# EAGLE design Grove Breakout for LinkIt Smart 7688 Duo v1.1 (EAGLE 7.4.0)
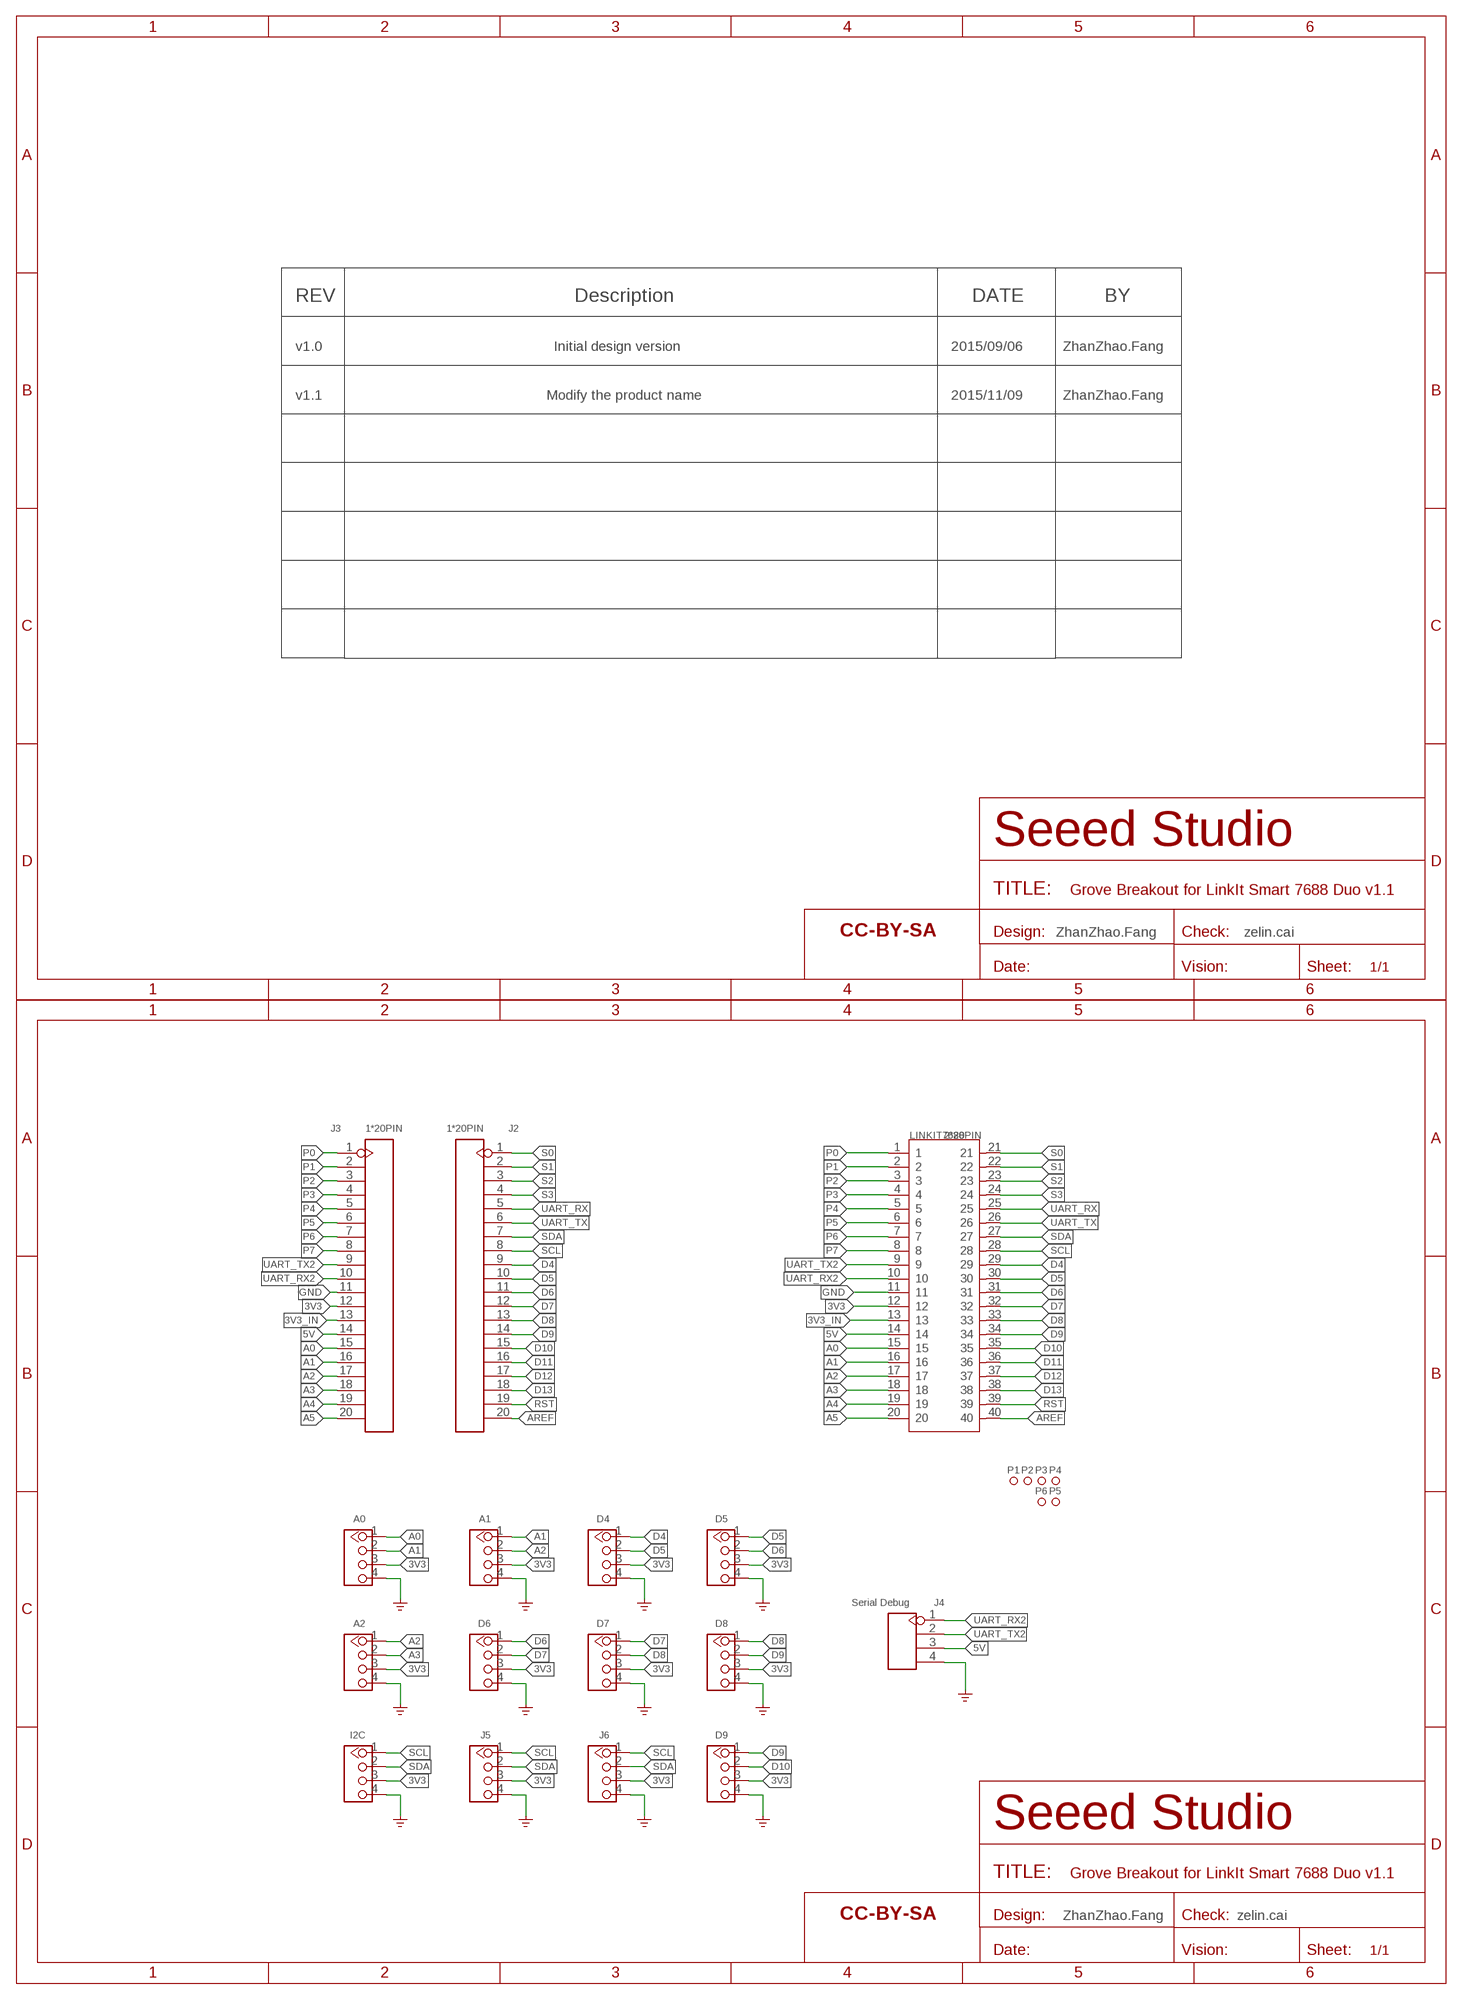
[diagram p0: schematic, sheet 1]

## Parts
A0  320110033  GROVE-CONNECTOR-DIP-2.0  [HW4-2.0]
A1  320110033  GROVE-CONNECTOR-DIP-2.0  [HW4-2.0]
A2  320110033  GROVE-CONNECTOR-DIP-2.0  [HW4-2.0]
D4  320110033  GROVE-CONNECTOR-DIP-2.0  [HW4-2.0]
D5  320110033  GROVE-CONNECTOR-DIP-2.0  [HW4-2.0]
D6  320110033  GROVE-CONNECTOR-DIP-2.0  [HW4-2.0]
D7  320110033  GROVE-CONNECTOR-DIP-2.0  [HW4-2.0]
D8  320110033  GROVE-CONNECTOR-DIP-2.0  [HW4-2.0]
D9  320110033  GROVE-CONNECTOR-DIP-2.0  [HW4-2.0]
FR1  DNP  SEEEDSTUDIO-OPEN-SCH-FRAME  [SEEEDSTUDIO-PCB-FRAME]
FR2  DNP  SEEEDSTUDIO-OPEN-SCH-FRAME  [SEEEDSTUDIO-PCB-FRAME]
I2C  320110033  GROVE-CONNECTOR-DIP-2.0  [HW4-2.0]
J2  1*20PIN  HEADER-20P-2.54  [H20-2.54]
J3  1*20PIN  HEADER-20P-2.54  [H20-2.54]
J4  Serial Debug  HEADER-4P-80/40MIL  [H4-2.54-C80D40MIL]
J5  320110033  GROVE-CONNECTOR-DIP-2.0  [HW4-2.0]
J6  320110033  GROVE-CONNECTOR-DIP-2.0  [HW4-2.0]
LINKIT7688  2*20PIN  LINKIT-7688-DUO  [HEADER-2X20P-2.54-65/35MIL]
P1  MARK-1.0'ANNULAR'  [ROUND-MARK-1.0]
P2  MARK-1.0'ANNULAR'  [ROUND-MARK-1.0]
P3  MARK-1.0'ANNULAR'  [ROUND-MARK-1.0]
P4  MARK-1.0'ANNULAR'  [ROUND-MARK-1.0]
P5  MARK-1.0'ANNULAR'  [ROUND-MARK-1.0]
P6  MARK-1.0'ANNULAR'  [ROUND-MARK-1.0]

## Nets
3V3: A0.3 A1.3 A2.3 D4.3 D5.3 D6.3 D7.3 D8.3 D9.3 I2C.3 J3.12 J5.3 J6.3 LINKIT7688.12
3V3_IN: J3.13 LINKIT7688.13
5V: J3.14 J4.3 LINKIT7688.14
A0: A0.1 J3.15 LINKIT7688.15
A1: A0.2 A1.1 J3.16 LINKIT7688.16
A2: A1.2 A2.1 J3.17 LINKIT7688.17
A3: A2.2 J3.18 LINKIT7688.18
A4: J3.19 LINKIT7688.19
A5: J3.20 LINKIT7688.20
AREF: J2.20 LINKIT7688.40
D4: D4.1 J2.9 LINKIT7688.29
D5: D4.2 D5.1 J2.10 LINKIT7688.30
D6: D5.2 D6.1 J2.11 LINKIT7688.31
D7: D6.2 D7.1 J2.12 LINKIT7688.32
D8: D7.2 D8.1 J2.13 LINKIT7688.33
D9: D8.2 D9.1 J2.14 LINKIT7688.34
D10: D9.2 J2.15 LINKIT7688.35
D11: J2.16 LINKIT7688.36
D12: J2.17 LINKIT7688.37
D13: J2.18 LINKIT7688.38
GND: A0.4 A1.4 A2.4 D4.4 D5.4 D6.4 D7.4 D8.4 D9.4 I2C.4 J3.11 J4.4 J5.4 J6.4 LINKIT7688.11 ; supply symbol labelled GND_POWER
P0: J3.1 LINKIT7688.1
P1: J3.2 LINKIT7688.2
P2: J3.3 LINKIT7688.3
P3: J3.4 LINKIT7688.4
P4: J3.5 LINKIT7688.5
P5: J3.6 LINKIT7688.6
P6: J3.7 LINKIT7688.7
P7: J3.8 LINKIT7688.8
RST: J2.19 LINKIT7688.39
S0: J2.1 LINKIT7688.21
S1: J2.2 LINKIT7688.22
S2: J2.3 LINKIT7688.23
S3: J2.4 LINKIT7688.24
SCL: I2C.1 J2.8 J5.1 J6.1 LINKIT7688.28
SDA: I2C.2 J2.7 J5.2 J6.2 LINKIT7688.27
UART_RX: J2.5 LINKIT7688.25
UART_RX2: J3.10 J4.1 LINKIT7688.10
UART_TX: J2.6 LINKIT7688.26
UART_TX2: J3.9 J4.2 LINKIT7688.9

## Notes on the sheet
- REV | Description | DATE | BY
- v1.0 | Initial design version | 2015/09/06 | ZhanZhao.Fang
- v1.1 | Modify the product name | 2015/11/09 | ZhanZhao.Fang
- ZhanZhao.Fang | zelin.cai
- ZhanZhao.Fang | zelin.cai

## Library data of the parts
A0 A1 A2 D4-D9 I2C J5 J6 = Connector-new:GROVE-CONNECTOR-DIP: 4P-2.0:320110033;4P-2.0-90D:320110034
FR1 FR2 = moudle-new:SEEEDSTUDIO-OPEN-SCH-FRAME
J2 J3 = Connector-new:HEADER-20P
J4 = Connector-new:HEADER-4P
LINKIT7688 = template:LINKIT-7688-DUO
P1-P6 = Discrete-new:MARK-1.0; PARTNO: DNP

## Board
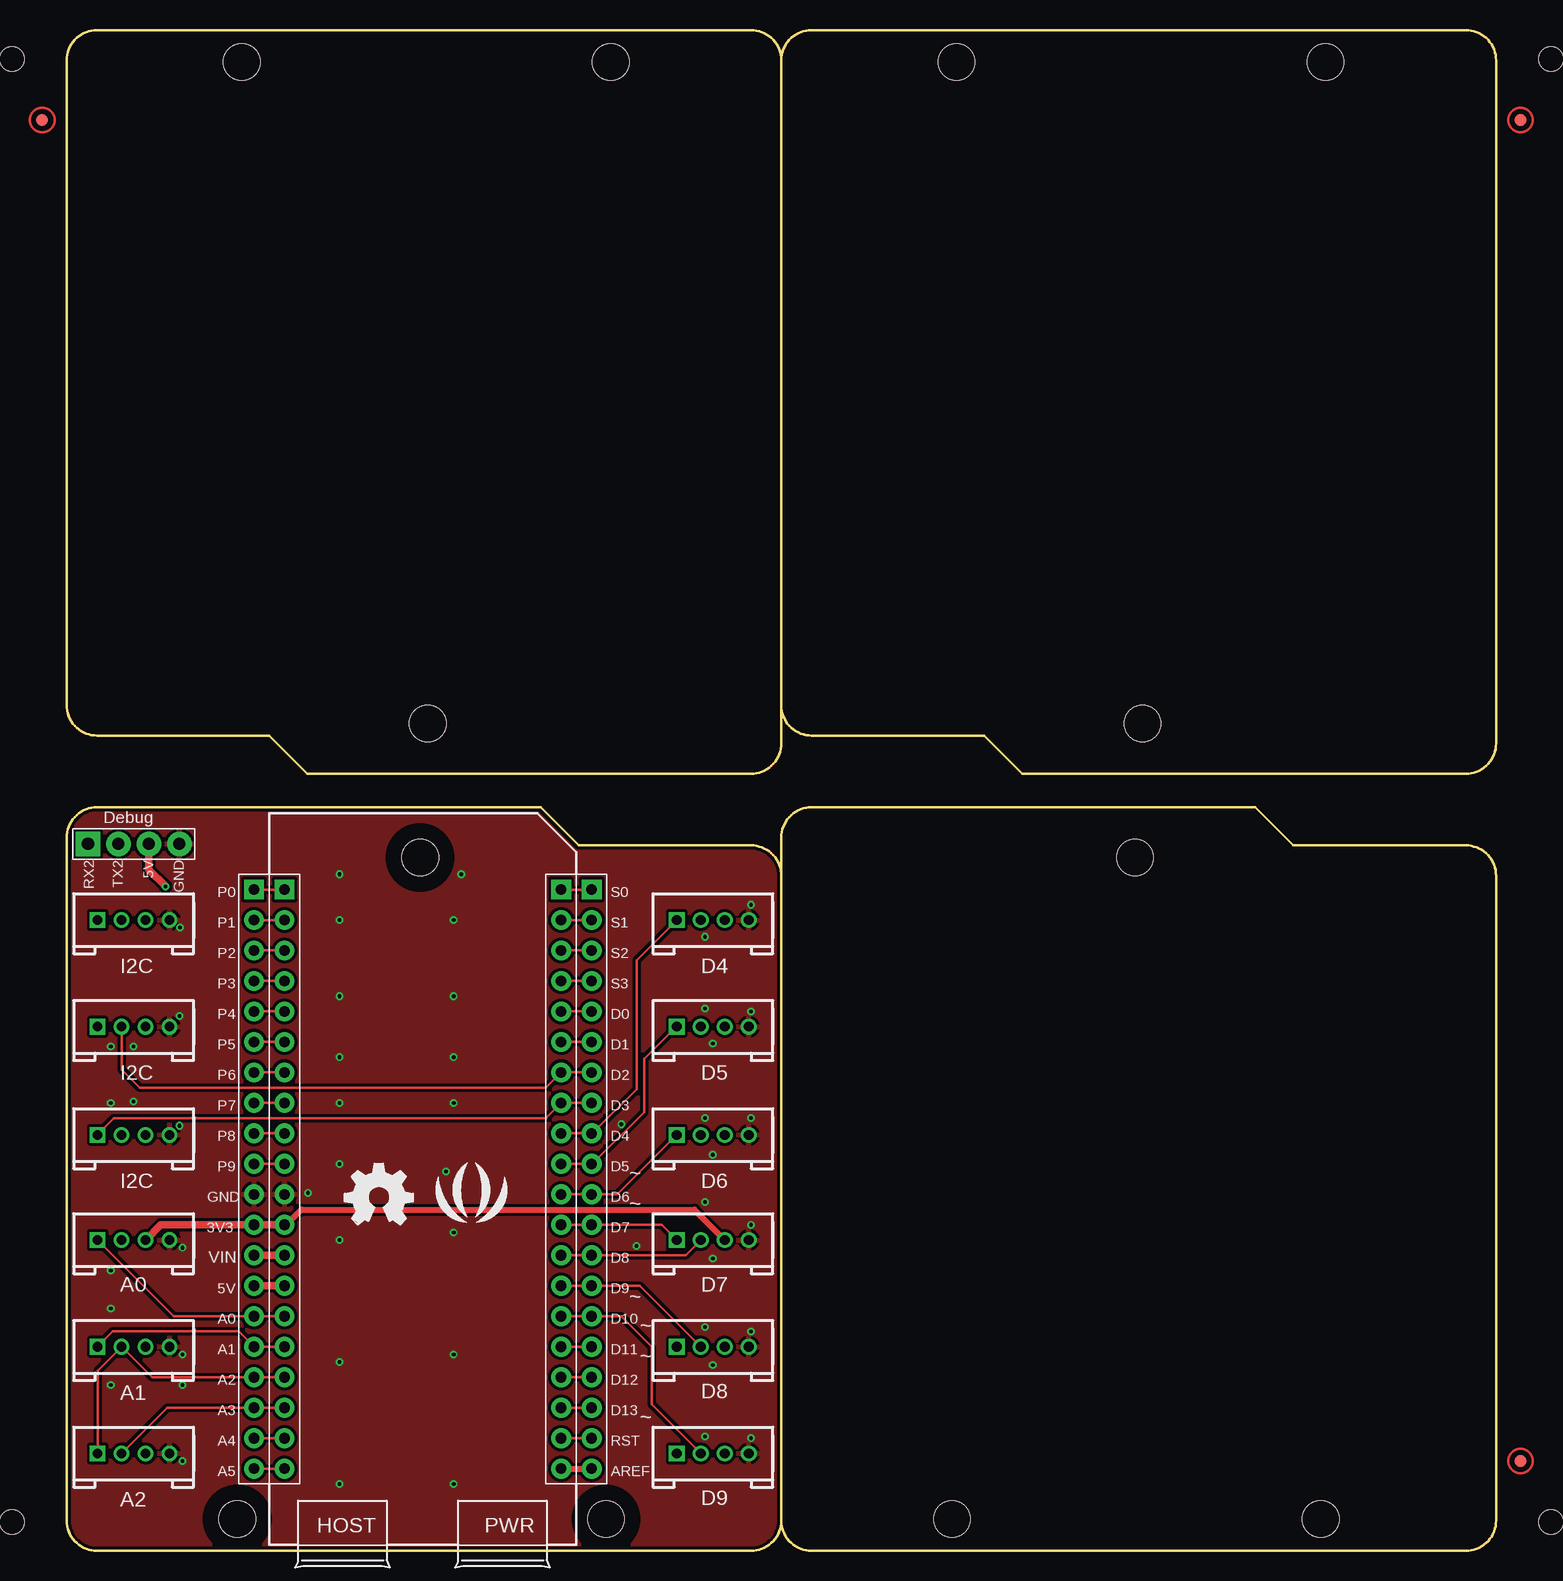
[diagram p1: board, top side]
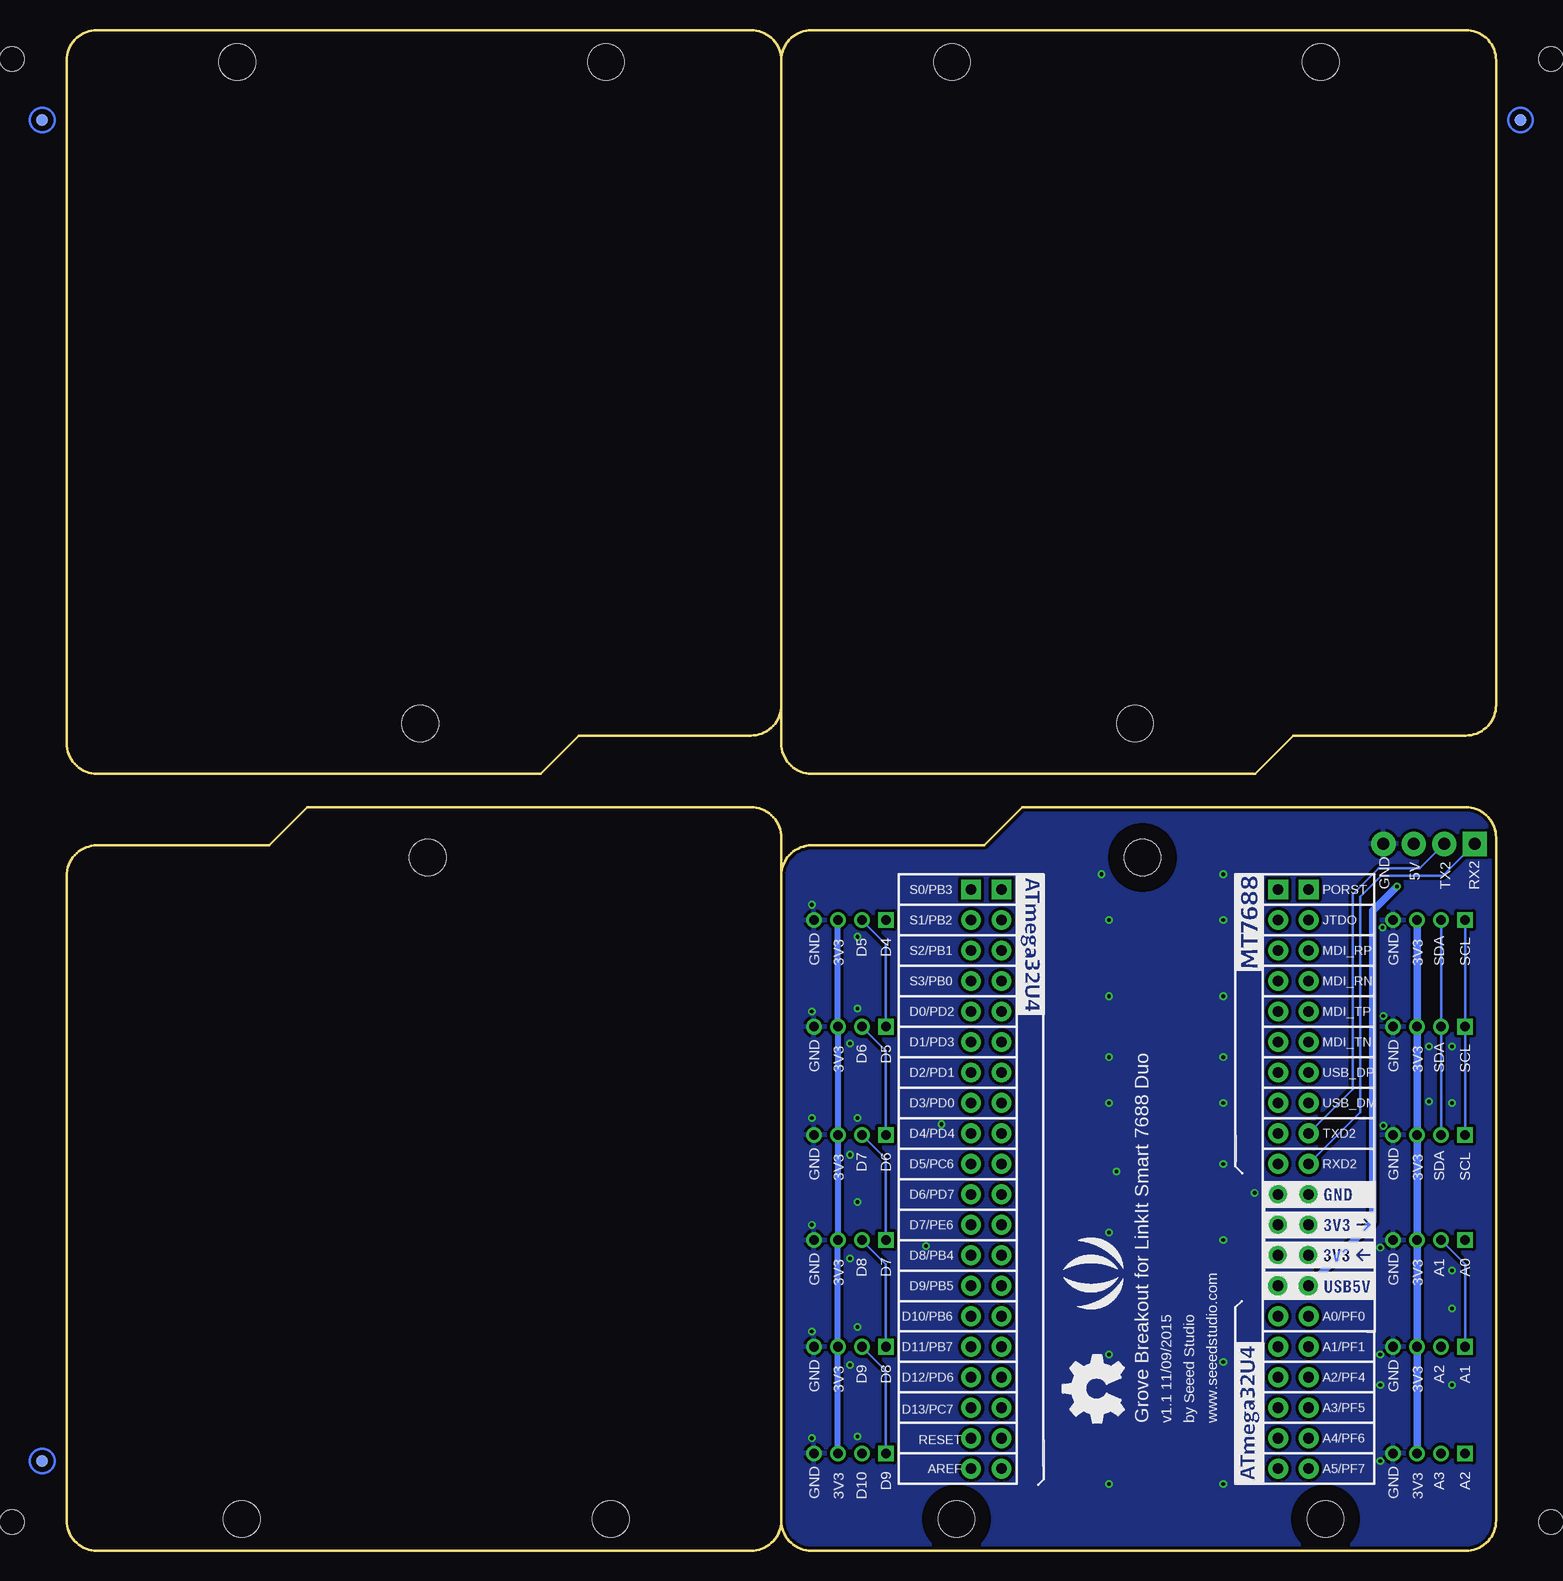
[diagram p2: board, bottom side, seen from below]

Size 119.13 x 126.75 mm. Coordinates in mm from the lower left corner, seen from the top.
Outline: 59.56,56.26 59.56,2.54
Outline: 59.56,2.54 arc-90 57.02,0 2.54,0 arc-90 0,2.54 0,59.44 arc-90 2.54,61.98 39.5,61.98 42.67,58.8 57.02,58.8 arc-90 59.56,56.26
Outline: 59.56,56.26 59.56,59.44 arc-90 62.1,61.98 99.06,61.98 102.23,58.8 116.59,58.8 arc-90 119.13,56.26 119.13,2.54 arc-90 116.59,0 62.1,0 arc-90 59.56,2.54
Outline: 59.56,70.48 59.56,124.21
Outline: 59.56,124.21 arc-90 62.1,126.75 116.59,126.75 arc-90 119.13,124.21 119.13,67.31 arc-90 116.59,64.77 79.63,64.77 76.45,67.94 62.1,67.94 arc-90 59.56,70.48
Outline: 59.56,70.48 59.56,67.31 arc-90 57.02,64.77 20.07,64.77 16.89,67.94 2.54,67.94 arc-90 0,70.48 0,124.21 arc-90 2.54,126.75 57.02,126.75 arc-90 59.56,124.21
Copper layers (1*16): Top 0.035mm / dielectric 1.5mm / Bottom 0.035mm
Design rules "SeeedStudio_2layer_DRU_no_angle_20140221 *": minimum track width 6mil, minimum drill 12mil, track to track 6mil, track to pad 6mil, pad to pad 6mil, via to via 6mil, smd to smd 0mil, copper to edge 10mil, drill to drill 10mil, minimum pad ring 10mil, minimum via ring 6mil, stop-mask expansion 2mil, vias tented up to drill 25mil, thermal gap 10mil
Holes 3.05 mm at 29.46,57.79 14.22,2.67 44.96,2.67 89.03,57.79 73.79,2.67 104.52,2.67 89.66,68.96 104.9,124.08 74.17,124.08 30.1,68.96 45.34,124.08 14.61,124.08
Holes 2.03 mm at -4.57,124.33 -4.57,2.41 123.7,124.33 123.7,2.41
tRestrict: area 27,55.3 to 32,60.3; area 11.7,0.2 to 16.7,5.2; area 42.5,0.2 to 47.5,5.2
bRestrict: area 27,55.3 to 32,60.3; area 11.7,0.2 to 16.7,5.2; area 42.5,0.2 to 47.5,5.2

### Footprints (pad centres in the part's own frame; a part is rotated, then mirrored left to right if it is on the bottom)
HW4-2.0 = drill 0.8 pad 1.27 square: 1 -3,0 | drill 0.8 pad 1.27: 2 -1,0; 3 1,0; 4 3,0
H20-2.54 = drill 0.889 pad 1.651 square: 1 0,-24.13 | drill 0.889 pad 1.651: 2 0,-21.59; 3 0,-19.05; 4 0,-16.51; 5 0,-13.97; 6 0,-11.43; 7 0,-8.89; 8 0,-6.35; 9 0,-3.81; 10 0,-1.27; 11 0,1.27; 12 0,3.81; 13 0,6.35; 14 0,8.89; 15 0,11.43; 16 0,13.97; 17 0,16.51; 18 0,19.05; 19 0,21.59; 20 0,24.13
H4-2.54-C80D40MIL = drill 1.016 pad 2.032 square: 1 0,3.81 | drill 1.016 pad 2.032: 2 0,1.27; 3 0,-1.27; 4 0,-3.81
HEADER-2X20P-2.54-65/35MIL = drill 0.889 pad 1.651 square: 1 0,24.13; 21 23.05,24.13 | drill 0.889 pad 1.651: 2 0,21.59; 3 0,19.05; 4 0,16.51; 5 0,13.97; 6 0,11.43; 7 0,8.89; 8 0,6.35; 9 0,3.81; 10 0,1.27; 11 0,-1.27; 12 0,-3.81; 13 0,-6.35; 14 0,-8.89; 15 0,-11.43; 16 0,-13.97; 17 0,-16.51; 18 0,-19.05; 19 0,-21.59; 20 0,-24.13; 22 23.05,21.59; 23 23.05,19.05; 24 23.05,16.51; 25 23.05,13.97; 26 23.05,11.43; 27 23.05,8.89; 28 23.05,6.35; 29 23.05,3.81; 30 23.05,1.27; 31 23.05,-1.27; 32 23.05,-3.81; 33 23.05,-6.35; 34 23.05,-8.89; 35 23.05,-11.43; 36 23.05,-13.97; 37 23.05,-16.51; 38 23.05,-19.05; 39 23.05,-21.59; 40 23.05,-24.13
ROUND-MARK-1.0 = smd 1.016 x 1.016: P$1 0,0

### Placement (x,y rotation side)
A0  5.59,25.91 0 top
A1  5.59,17.02 0 top
A2  5.59,8.13 0 top
D4  53.85,52.58 0 top
D5  53.85,43.69 0 top
D6  53.85,34.67 0 top
D7  53.85,25.91 0 top
D8  53.85,17.02 0 top
D9  53.85,8.13 0 top
FR1  not placed on the board
FR2  not placed on the board
I2C  5.59,52.58 0 top
J2  43.75,30.99 180 top
J3  15.62,30.99 180 top
J4  5.59,58.93 90 top
J5  5.59,43.69 0 top
J6  5.59,34.67 0 top
LINKIT7688  18.16,30.99 0 top
P1  -2.03,119.25 0 top
P2  -2.03,119.25 0 bottom
P3  121.16,119.25 0 top
P4  121.16,119.25 0 bottom
P5  121.16,7.49 0 top
P6  121.16,7.49 0 bottom
U$14  [OSHW_FILLX200_NOTEXT]  31.01,10.68 90 bottom
U$15  [SEEED-SILK-280*268MIL]  32.77,23.11 90 bottom
U$16  [OSHW_FILLX200_NOTEXT]  23.19,27.2 0 top
U$17  [SEEED-SILK-280*268MIL]  33.73,29.08 0 top

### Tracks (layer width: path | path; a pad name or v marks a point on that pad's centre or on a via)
3V3
  Top 0.508: LINKIT7688.12 18.29,27.18 19.56,28.45 52.31,28.45 D7.3
  Top 0.61: A0.3 7.86,27.18 J3.12 LINKIT7688.12
  Bottom 0.508: D9.3 D8.3 D7.3 D6.3 D5.3 D4.3
  Bottom 0.61: A2.3 A1.3 A0.3 J6.3 J5.3 I2C.3
3V3_IN
  Top 0.61: J3.13 LINKIT7688.13
5V  (via drill 0.3 pad 0.64)
  Top 0.61: J3.14 LINKIT7688.14 | J4.3 6.86,56.77 v8.26,55.37
  Bottom 0.61: v8.26,55.37 10.29,53.34 10.29,27.43 J3.14
A0
  Top 0.203: A0.1 8.94,19.56 J3.15 LINKIT7688.15
A1
  Top 0.203: LINKIT7688.16 J3.16 14.35,18.29 3.86,18.29 A1.1
  Bottom 0.203: A1.1 2.59,23.91 A0.2
A2
  Top 0.203: A2.1 2.59,15.02 A1.2 7.13,14.48 J3.17 LINKIT7688.17
A3
  Top 0.203: A2.2 8.4,11.94 J3.18 LINKIT7688.18
A4
  Top 0.203: J3.19 LINKIT7688.19
A5
  Top 0.203: J3.20 LINKIT7688.20
AREF
  Top 0.508: LINKIT7688.40 J2.20
D4
  Top 0.203: LINKIT7688.29 J2.9 43.81,34.8 47.5,38.48 47.5,49.23 D4.1
D5
  Top 0.203: LINKIT7688.30 J2.10 43.81,32.26 48.13,36.58 48.13,41.02 50.8,43.69 D5.1
  Bottom 0.203: D5.1 50.85,50.58 D4.2
D6
  Top 0.203: LINKIT7688.31 J2.11 45.9,29.72 D6.1
  Bottom 0.203: D6.1 50.85,41.69 D5.2
D7
  Top 0.203: LINKIT7688.32 J2.12 49.58,27.18 D7.1
  Bottom 0.203: D7.1 50.85,32.67 D6.2
D8
  Top 0.203: LINKIT7688.33 J2.13 51.58,24.64 D7.2
  Bottom 0.203: D8.1 50.85,23.91 D7.2
D9
  Top 0.203: LINKIT7688.34 J2.14 47.77,22.1 D8.2
  Bottom 0.203: D9.1 50.85,15.02 D8.2
D10
  Top 0.203: LINKIT7688.35 J2.15 46.23,19.56 48.77,17.02 48.77,12.21 D9.2
D11
  Top 0.203: LINKIT7688.36 J2.16
D12
  Top 0.203: LINKIT7688.37 J2.17
D13
  Top 0.203: LINKIT7688.38 J2.18
GND  (via drill 0.3 pad 0.64)
  other vias: 9.46,51.94 9.4,44.58 9.4,35.43 9.65,25.27 9.65,16.38 9.65,7.49 20.12,29.84 57.02,9.4 57.02,18.29 57.02,27.18 57.02,36.07 57.02,44.96 57.02,53.85 22.73,5.59 32.26,5.59 32.26,16.38 22.73,15.75 22.73,25.91 32.26,26.54 32.26,41.15 22.73,41.15 22.73,56.39 32.89,56.39 31.62,31.62 22.73,32.26 22.73,46.23 32.26,46.23 22.73,37.34 32.26,37.34 3.68,13.84 9.65,13.84 22.73,52.58 32.26,52.58 46.23,35.56 47.5,25.4 53.21,51.18 53.21,45.21 53.85,42.29 53.21,36.07 53.85,33.02 53.21,29.08 53.85,24.38 53.21,18.67 53.85,15.49 53.21,9.52 3.68,20.19 3.68,23.37 3.68,37.34 3.68,42.04 5.59,42.04 5.59,37.47
  pour Bottom (isolate 0.254): -0.63,62.74 60.2,62.74 60.2,-0.76 -0.63,-0.76
  pour Top (isolate 0.254): -0.63,62.74 60.2,62.74 60.2,-0.76 -0.63,-0.76
P0
  Top 0.203: J3.1 LINKIT7688.1
P1
  Top 0.203: J3.2 LINKIT7688.2
P2
  Top 0.203: J3.3 LINKIT7688.3
P3
  Top 0.203: J3.4 LINKIT7688.4
P4
  Top 0.203: J3.5 LINKIT7688.5
P5
  Top 0.203: J3.6 LINKIT7688.6
P6
  Top 0.203: J3.7 LINKIT7688.7
P7
  Top 0.203: J3.8 LINKIT7688.8
RST
  Top 0.203: LINKIT7688.39 J2.19
S0
  Top 0.203: LINKIT7688.21 J2.1
S1
  Top 0.203: LINKIT7688.22 J2.2
S2
  Top 0.203: J2.3 LINKIT7688.23
S3
  Top 0.203: LINKIT7688.24 J2.4
SCL
  Top 0.203: J6.1 2.59,34.72 3.94,36.07 39.94,36.07 LINKIT7688.28 J2.8
  Bottom 0.203: J6.1 J5.1 I2C.1
SDA
  Top 0.203: J5.2 4.59,40.12 6.1,38.61 39.94,38.61 LINKIT7688.27 J2.7
  Bottom 0.203: J6.2 J5.2 I2C.2
UART_RX
  Top 0.203: LINKIT7688.25 J2.5
UART_RX2
  Top 0.203: LINKIT7688.10 J3.10
  Bottom 0.203: J3.10 11.3,36.58 11.3,54.53 9.58,56.26 4.45,56.26 J4.1
UART_TX
  Top 0.203: LINKIT7688.26 J2.6
UART_TX2
  Top 0.203: J3.9 LINKIT7688.9
  Bottom 0.203: J3.9 11.94,38.48 11.94,54.74 9.78,56.9 6.35,56.9 J4.2

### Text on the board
tPlace: Debug | RX2 | TX2 | 5V | GND | P0 | S0 | P1 | S1 | P2 | S2 | P3 | S3 | P4 | D0 | P5 | D1 | I2C | P6 | D2 | P7 | D3 | P8 | D4 | P9 | D5 | I2C | ~ | GND | D6 | ~ | 3V3 | D7 | VIN | D8 | 5V | D9 | ~ | A0 | D10 | ~ | A1 | D11 | ~ | A2 | D12 | A3 | D13 | ~ | A4 | RST | A5 | AREF | HOST | PWR
bPlace: RX2 | TX2 | 5V | GND | PORST | S0/PB3 | JTDO | S1/PB2 | MDI_RP | S2/PB1 | D4 | D5 | SCL | SDA | 3V3 | GND | 3V3 | GND | MDI_RN | S3/PB0 | MDI_TP | D0/PD2 | MDI_TN | D1/PD3 | D5 | D6 | SCL | SDA | 3V3 | GND | USB_DP | D2/PD1 | 3V3 | GND | USB_DM | D3/PD0 | TXD2 | D4/PD4 | RXD2 | D5/PC6 | D6 | D7 | SCL | SDA | 3V3 | GND | 3V3 | GND | D6/PD7 | D7/PE6 | D8/PB4 | A0 | A1 | 3V3 | GND | D7 | D8 | 3V3 | GND | D9/PB5 | A0/PF0 | D10/PB6 | A1/PF1 | D11/PB7 | A2/PF4 | D12/PD6 | A1 | A2 | 3V3 | GND | D8 | D9 | 3V3 | GND | A3/PF5 | D13/PC7 | www.seeedstudio.com | by Seeed Studio | v1.1 11/09/2015 | Grove Breakout for LinkIt Smart 7688 Duo | A4/PF6 | RESET | A5/PF7 | AREF | A2 | A3 | D9 | 3V3 | GND | D10 | 3V3 | GND

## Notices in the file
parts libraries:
moudle-new: This work is licensed under the Creative Commons Attribution 4.0 International License.
To view a copy of this license,visit:
http://creativecommons.org/licenses/by-sa/4.0
moudle-new: CC-BY-SA
